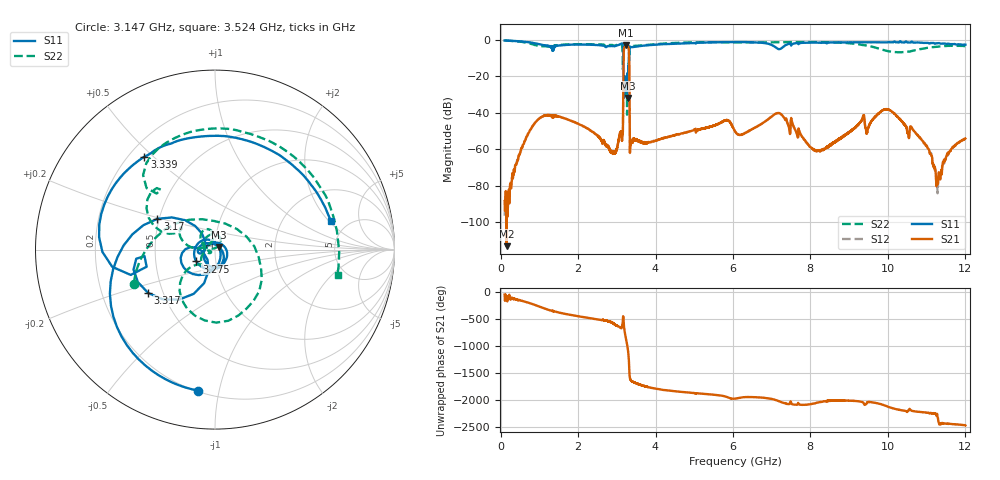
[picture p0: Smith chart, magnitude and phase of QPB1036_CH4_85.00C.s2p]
! TDS: K:\Engsetup\Winsaw\QPB1036_ALL
! Channel 1
! Ports=1 2
! seg 1=100.000000 1100.000000 101
! seg 2=1101.000000 1501.000000 401
! seg 3=1502.000000 2502.000000 101
! seg 4=2503.000000 3803.000000 1301
! seg 5=3804.000000 5004.000000 121
! seg 6=5005.000000 6005.000000 1001
! seg 7=6006.000000 8406.000000 241
! seg 8=8407.000000 10607.000000 2201
! seg 9=10608.000000 12008.000000 141
! Points=5609
! FailCode=0
! Topology=ALL_SE(12)
!VNA Cal loaded =QPB1036_ALL_85C
!PS1(V)= 5.000
!PS(mA)= 0.500
!PS2(V)= 1.170
!PS(mA)= -0.100
!PS3(V)= 0.630
!PS(mA)= 0.100
!PS4(V)= 0.630
!PS(mA)= -0.100
!Temp (C)= 85.00
# MHz S DB R 50
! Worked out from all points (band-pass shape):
!   5609 points, 100 MHz to 12.01 GHz, reference 50 ohm
!   highest |S21| = -2.98 dB at 3.227 GHz (marker M1); lowest = -113.1 dB at 150 MHz (marker M2)
!   |S21| within 3 dB of the highest: 3.181 GHz to 3.312 GHz (131.3 MHz wide, 4.05 % of centre)
!   lowest |S11| = -31.9 dB at 3.291 GHz (marker M3), VSWR 1.05, Z = 52.1 + j1.55 ohm
!   |S11| at or under -10 dB: 3.171 GHz to 3.315 GHz (143.9 MHz wide, 4.44 % of centre)
!   |S22| runs from -41.0 to -0.3 dB; largest |S21 - S12| = 0.0087
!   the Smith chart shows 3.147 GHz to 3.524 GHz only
!   S11 on the Smith chart (normalised r, x): 3.147 GHz: 0.21, -0.86; 3.17 GHz: 0.49, +0.19; 3.275 GHz: 0.80, -0.11; 3.317 GHz: 0.41, -0.25; 3.339 GHz: 0.26, +0.47; 3.524 GHz: 3.67, +2.11
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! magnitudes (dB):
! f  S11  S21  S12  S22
! 100 MHz  -0.3  -88.4  -96.4  -0.3
! 150 MHz  -0.4  -113.1  -95.0  -0.4
! 1.124 GHz  -2.9  -41.7  -41.7  -3.5
! 2.092 GHz  -2.5  -46.9  -47.0  -2.3
! 2.921 GHz  -3.4  -62.1  -61.8  -3.1
! 3.147 GHz  -2.0  -50.8  -50.6  -6.2
! 3.17 GHz  -8.8  -16.5  -16.5  -8.0
! 3.195 GHz  -26.3  -3.9  -3.9  -20.3
! 3.227 GHz  -21.2  -3.0  -2.9  -26.2
! 3.275 GHz  -18.2  -3.3  -3.3  -21.3
! 3.291 GHz  -31.9  -3.8  -3.7  -22.1
! 3.317 GHz  -7.1  -9.1  -9.1  -7.0
! 3.339 GHz  -3.7  -61.9  -62.0  -3.4
! 3.36 GHz  -4.0  -56.1  -56.5  -3.4
! 3.524 GHz  -3.6  -55.3  -55.2  -3.1
! 4.074 GHz  -2.5  -54.9  -54.8  -2.2
! 6.056 GHz  -1.2  -50.1  -50.2  -1.3
! 7.146 GHz  -4.7  -40.2  -40.1  -1.3
! 8.046 GHz  -1.5  -59.3  -59.5  -1.1
! 10.02 GHz  -1.1  -38.1  -38.2  -6.2
! 11.28 GHz  -1.8  -78.4  -78.5  -3.7
! 12.01 GHz  -2.6  -54.1  -54.0  -3.4
